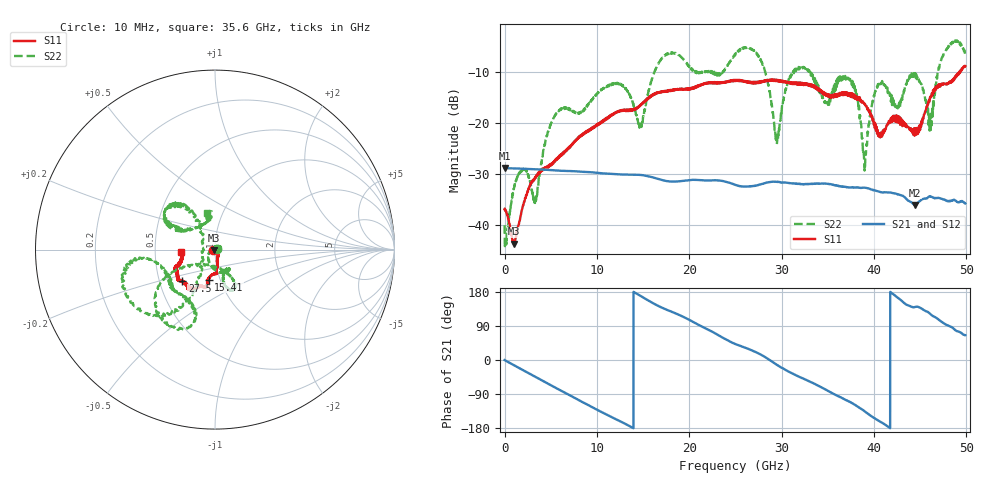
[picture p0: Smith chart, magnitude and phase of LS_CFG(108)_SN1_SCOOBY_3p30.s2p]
!Keysight Technologies,N5245B,MY58422026,A.13.80.08
!Date: Friday, March 20, 2020 00:01:03
!Correction: S11(Full 2 Port(1,2))
!S21(Full 2 Port(1,2))
!S12(Full 2 Port(1,2))
!S22(Full 2 Port(1,2))
!S2P File: Measurements: S11, S21, S12, S22:
# Hz S DB R 50.0
!freq dBS11 angS11 dBS21 angS21 dBS12 angS12 dBS22 angS22
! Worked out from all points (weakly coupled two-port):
!   4991 points, 10 MHz to 49.91 GHz, reference 50 ohm
!   highest |S21| = -28.86 dB at 30 MHz (marker M1); lowest = -36.2 dB at 44.44 GHz (marker M2)
!   lowest |S11| = -43.8 dB at 990 MHz (marker M3), VSWR 1.01, Z = 49.5 - j0.442 ohm
!   |S11| at or under -10 dB: start of sweep to 49.24 GHz; 49.29704 GHz to 49.33355 GHz (36.51 MHz wide, 0.074 % of centre)
!   |S22| runs from -44.3 to -3.7 dB; largest |S21 - S12| = 0.00036
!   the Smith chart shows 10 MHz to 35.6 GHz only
!   S11 on the Smith chart (normalised r, x): 10 MHz: 0.97, -0.01; 15.41 GHz: 0.88, -0.30; 27.5 GHz: 0.65, -0.25; 35.6 GHz: 0.68, -0.02
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1e7  -36.97 -168.3  -28.86 -0.2  -28.84 -0.3  -40.13 4.9
3e7  -36.88 -179.4  -28.86 -0.4  -28.85 -0.5  -43.32 -10.6
9.9e8  -43.78 -136.4  -28.93 -13.3  -28.93 -13.3  -32.96 -32.9
3.31e9  -30.66 -58.6  -29.10 -43.9  -29.10 -43.9  -35.36 130.4
5.37e9  -27.45 -67.5  -29.29 -71.2  -29.29 -71.2  -18.83 -88.4
8.33e9  -22.53 -80.3  -29.57 -109.7  -29.56 -109.6  -17.79 -63.8
1.541e10  -15.38 -101.8  -30.41 159.4  -30.41 159.5  -15.37 -147.0
1.665e10  -14.03 -102.1  -31.02 142.8  -31.01 142.9  -8.29 -145.5
2.496e10  -11.65 -124.8  -32.13 42.6  -32.12 42.8  -6.56 -170.9
2.75e10  -11.91 -135.9  -32.20 17.4  -32.22 17.8  -6.66 -127.6
2.948e10  -11.52 -140.6  -31.56 -12.4  -31.56 -12.0  -23.89 -177.3
3.103e10  -12.01 -147.7  -31.87 -34.0  -31.87 -33.8  -10.40 125.8
3.328e10  -12.58 -157.6  -31.98 -59.6  -31.97 -59.3  -10.61 153.2
3.56e10  -14.43 -174.8  -32.20 -89.1  -32.13 -88.7  -13.90 101.6
3.77e10  -14.92 175.2  -32.67 -114.8  -32.60 -114.9  -12.16 131.6
3.902e10  -16.22 173.1  -32.72 -135.7  -32.70 -135.9  -28.57 -114.6
4.021e10  -21.30 162.7  -33.36 -155.8  -33.32 -156.0  -13.46 -8.7
4.16e10  -19.71 106.2  -33.67 -177.1  -33.70 -177.2  -14.14 22.6
4.444e10  -21.96 54.0  -36.15 139.8  -36.18 140.1  -10.57 -18.2
4.614e10  -14.85 6.8  -34.42 120.5  -34.45 120.6  -21.43 -50.7
4.757e10  -12.20 7.0  -35.08 96.9  -35.09 97.0  -6.27 -80.2
4.991e10  -8.75 -12.6  -35.82 65.4  -35.86 65.6  -6.27 -28.6
